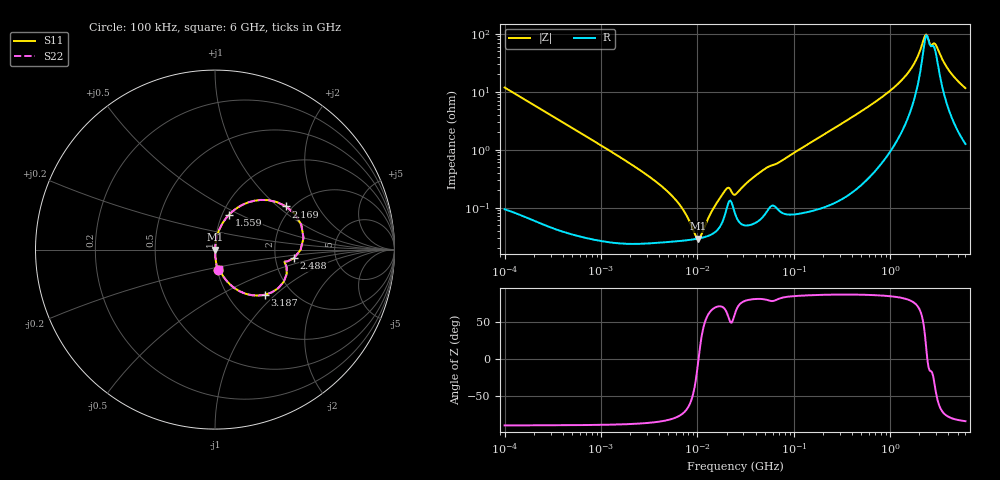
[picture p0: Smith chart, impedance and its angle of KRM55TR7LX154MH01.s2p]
!Murata Part Number: KRM55TR7LX154MH01
!These Parameters are Measured in Series Mode Connection
!Data Generated on Jan 08, 2026
!  o--ll--o
!Port1  Port2
!  o------o
!Operation Temp=25[degC], DC Bias Voltage=0[V]
!Freq. Start=100[kHz] Stop=6[GHz] 401[Steps]
# Hz S RI R 50
!Freq.(Hz) S11(Real) S11(Imag) S21(Real) S21(Imag) S12(Real) S12(Imag) S22(Real) S22(Imag)
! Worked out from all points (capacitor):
!   401 points, 100 kHz to 6 GHz, reference 50 ohm
!   read as one part in series: C = 135 nF near 105.7 kHz
!   lowest |Z| = 29.1 mohm at 10.16 MHz (marker M1)
!   series resonance near 10.25 MHz, so ESL is about 1.8 nH
!   S11 on the Smith chart (normalised r, x): 100 kHz: 1.00, -0.24; 1.559 GHz: 1.08, +0.44; 2.169 GHz: 1.86, +1.14; 2.488 GHz: 2.54, -0.30; 3.187 GHz: 1.47, -0.86; 6 GHz: 1.03, -0.23
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100000  0.0146 -0.1162  0.9854 0.1162  0.9854 0.1162  0.0146 -0.1162
631452  0.000662 -0.0188  0.9993 0.0188  0.9993 0.0188  0.000662 -0.0188
3987316  0.000253 -0.00253  0.9997 0.00253  0.9997 0.00253  0.000253 -0.00253
6541803  0.000265 -0.00108  0.9997 0.00108  0.9997 0.00108  0.000265 -0.00108
1.015836e7  0.00029 -2.05e-05  0.9997 2.05e-05  0.9997 2.05e-05  0.00029 -2.05e-05
1.103214e7  0.000299 0.000176  0.9997 -0.000176  0.9997 -0.000176  0.000299 0.000176
1.452491e7  0.000356 0.000876  0.9996 -0.000876  0.9996 -0.000876  0.000356 0.000876
1.965679e7  0.000843 0.00185  0.9992 -0.00185  0.9992 -0.00185  0.000843 0.00185
2.076842e7  0.00117 0.00186  0.9988 -0.00186  0.9988 -0.00186  0.00117 0.00186
2.517799e7  0.000699 0.00157  0.9993 -0.00157  0.9993 -0.00157  0.000699 0.00157
4.872031e7  0.000736 0.00445  0.9993 -0.00445  0.9993 -0.00445  0.000736 0.00445
1.546735e8  0.00106 0.0137  0.9989 -0.0137  0.9989 -0.0137  0.00106 0.0137
9.76689e8  0.0186 0.0982  0.9814 -0.0982  0.9814 -0.0982  0.0186 0.0982
1.558934e9  0.0785 0.1943  0.9215 -0.1943  0.9215 -0.1943  0.0785 0.1943
1.889928e9  0.1894 0.2645  0.8106 -0.2645  0.8106 -0.2645  0.1894 0.2645
2.168564e9  0.3957 0.2407  0.6043 -0.2407  0.6043 -0.2407  0.3957 0.2407
2.2912e9  0.481 0.1376  0.519 -0.1376  0.519 -0.1376  0.481 0.1376
2.488279e9  0.4396 -0.0479  0.5604 0.0479  0.5604 0.0479  0.4396 -0.0479
2.934752e9  0.3835 -0.1783  0.6165 0.1783  0.6165 0.1783  0.3835 -0.1783
3.187187e9  0.2776 -0.2517  0.7224 0.2517  0.7224 0.2517  0.2776 -0.2517
3.971646e9  0.0966 -0.2052  0.9034 0.2052  0.9034 0.2052  0.0966 -0.2052
6e9  0.0248 -0.1103  0.9752 0.1103  0.9752 0.1103  0.0248 -0.1103
